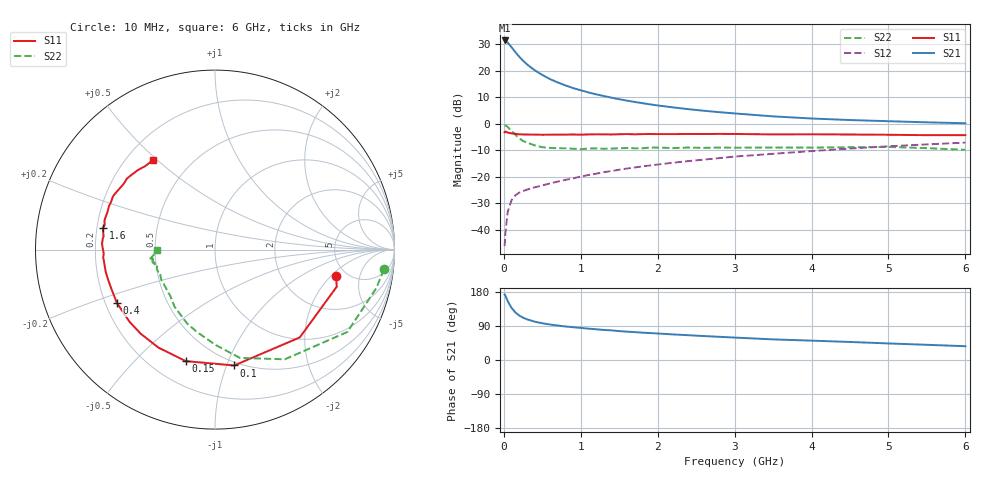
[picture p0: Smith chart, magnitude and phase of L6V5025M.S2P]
!  INFINEON TECHNOLOGIES Small Signal Semiconductors
! BFR380L3 , Si-NPN RF-Transistor in TSLP-3-1
!  Vce=0.5 V,  Ic=25 mA
! Common Emitter S-Parameters:  07. March 2005
#  GHz  S  MA  R  50
! f  S11  S21  S12  S22
! GHz  Mag  Ang  Mag  Ang  Mag  Ang  Mag  Ang
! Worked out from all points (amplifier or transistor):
!   36 points, 10 MHz to 6 GHz, reference 50 ohm
!   highest |S21| = 31.4 dB at 10 MHz (marker M1)
!   |S21| within 3 dB of that: start of sweep to 112.2 MHz
!   unconditionally stable (mu >= 1): 1.342 GHz to end of sweep
!   at 250 MHz: K = 0.44, MSG = 24.6 dB, |S12| = -25.4 dB
!   at 1.4 GHz: K = 1.01, MAG = 13.3 dB, |S12| = -17.9 dB
!   at 6 GHz: K = 1.01, MAG = 3.1 dB, |S12| = -7.2 dB
!   S11 on the Smith chart (normalised r, x): 10 MHz: 4.11, -2.28; 100 MHz: 0.47, -1.06; 150 MHz: 0.34, -0.71; 400 MHz: 0.25, -0.24; 1.6 GHz: 0.22, +0.09; 6 GHz: 0.31, +0.48
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0.01  0.689 -12.2  37.01 173.0  0.0049 78.2  0.9474 -6.7
0.02  0.7092 -16.9  36.45 169.9  0.0086 83.9  0.9243 -13.4
0.05  0.6801 -46.0  33.76 155.5  0.0216 70.3  0.8685 -31.9
0.1  0.6544 -80.6  27.61 137.6  0.0361 57.5  0.7246 -57.5
0.15  0.6424 -104.7  22.26 125.4  0.0446 49.6  0.6195 -77.0
0.2  0.6305 -119.9  18.27 117.4  0.0501 46.4  0.5311 -89.7
0.25  0.6253 -131.3  15.38 111.7  0.0535 44.0  0.4704 -102.2
0.3  0.6234 -139.6  13.13 107.4  0.057 44.3  0.4403 -110.6
0.4  0.6222 -151.5  10.18 101.2  0.063 45.2  0.39 -125.3
0.5  0.6173 -159.1  8.279 97.0  0.0685 47.3  0.3595 -133.6
0.6  0.6189 -164.5  6.916 93.6  0.0748 49.2  0.3491 -140.4
0.7  0.6215 -168.6  5.987 91.0  0.0808 51.2  0.3436 -146.4
0.9  0.6244 -176.1  4.684 86.5  0.0929 54.4  0.3367 -154.8
1.1  0.6261 179.2  3.881 82.7  0.1076 56.7  0.3397 -158.3
1.3  0.6281 174.3  3.317 79.3  0.1217 58.1  0.3365 -163.9
1.6  0.6356 168.9  2.716 74.8  0.1425 59.3  0.3472 -167.4
2.2  0.6347 160.5  2.025 67.5  0.1835 60.6  0.3464 -169.2
2.8  0.6407 152.6  1.646 61.2  0.224 60.8  0.3537 -172.5
3.5  0.6271 144.5  1.372 54.4  0.2701 58.7  0.3547 -172.3
4.5  0.6241 138.1  1.17 47.6  0.3396 56.5  0.3592 -172.4
5.5  0.606 129.8  1.059 40.1  0.4065 51.9  0.3453 -174.6
6  0.6068 124.7  1.017 36.4  0.439 49.5  0.3209 -179.6
